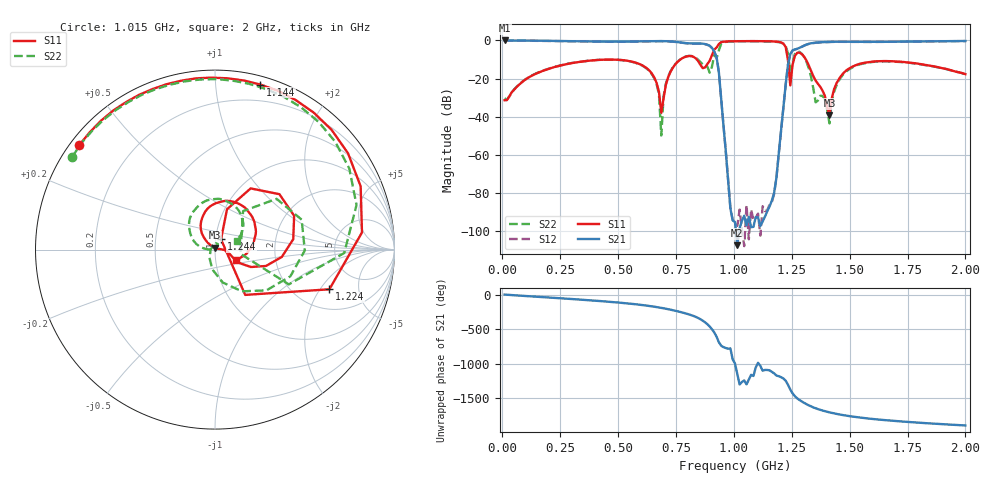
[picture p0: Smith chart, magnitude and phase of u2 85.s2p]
!Agilent Technologies,E8363B,SG43030131,A.07.50.48
!Agilent E8363B: A.07.50.48
!Date: Tuesday, December 02, 2025 02:39:29
!Correction: S11(Full 2 Port(1,2))
!S21(Full 2 Port(1,2))
!S12(Full 2 Port(1,2))
!S22(Full 2 Port(1,2))
!S2P File: Measurements: S11, S21, S12, S22:
# Hz S  dB  R 50
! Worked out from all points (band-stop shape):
!   201 points, 10 MHz to 2 GHz, reference 50 ohm
!   highest |S21| = -0.01 dB at 10 MHz (marker M1); lowest = -107.4 dB at 1.015 GHz (marker M2)
!   |S21| within 3 dB of the highest: start of sweep to 897.6 MHz; 1.298 GHz to end of sweep
!   lowest |S11| = -39.3 dB at 1.413 GHz (marker M3), VSWR 1.02, Z = 49.8 + j1.07 ohm
!   |S11| at or under -10 dB: start of sweep to 769.2 MHz; 839.9 MHz to 897.7 MHz (57.8 MHz wide, 6.65 % of centre); 1.311 GHz to end of sweep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
!   |S22| runs from -49.9 to -0.4 dB; largest |S21 - S12| = 0.028
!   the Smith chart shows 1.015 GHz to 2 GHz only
!   S11 on the Smith chart (normalised r, x): 1.015 GHz: 0.03, +0.34; 1.144 GHz: 0.06, +1.31; 1.224 GHz: 3.02, -2.45; 1.244 GHz: 1.06, +0.12; 2 GHz: 1.25, -0.15
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1e7  -31.35 -84.1  -0.01 -0.2  -0.08 -1.8  -30.31 -82.0
3.483e8  -11.00 -166.0  -0.48 -76.0  -0.56 -76.1  -10.98 -163.0
6.7665e8  -26.97 90.9  -0.33 173.4  -0.40 173.2  -28.39 86.0
6.866e8  -37.97 119.2  -0.34 167.5  -0.40 167.5  -49.85 63.0
6.9655e8  -30.37 -131.6  -0.36 161.5  -0.42 161.4  -29.29 -103.2
7.264e8  -16.44 -138.1  -0.51 141.4  -0.58 141.3  -16.21 -123.5
8.5575e8  -12.78 57.2  -1.60 3.4  -1.67 3.2  -11.41 141.5
8.856e8  -12.44 -74.1  -2.25 -68.4  -2.30 -68.6  -13.63 125.3
9.1545e8  -4.79 -116.6  -5.87 172.2  -5.93 172.0  -7.67 -104.3
9.7515e8  -0.49 169.0  -73.45 -62.2  -72.79 -47.4  -0.63 176.2
1.005e9  -0.42 148.3  -95.23 83.7  -94.76 66.1  -0.47 153.2
1.01495e9  -0.40 142.5  -107.36 -69.8  -97.25 142.5  -0.45 147.0
1.1443e9  -0.41 74.6  -89.59 -9.3  -89.12 -89.0  -0.51 78.5
1.17415e9  -0.53 54.3  -79.77 -59.0  -80.40 -41.9  -0.66 58.9
1.2239e9  -3.42 -19.1  -23.12 -164.7  -23.18 -164.9  -2.85 -1.5
1.2438e9  -23.57 59.6  -7.14 68.5  -7.19 68.4  -16.85 -9.4
1.29355e9  -7.13 7.6  -3.27 -104.8  -3.34 -104.9  -7.03 -19.6
1.3433e9  -18.78 -25.3  -1.30 170.6  -1.37 170.5  -25.20 -124.3
1.41295e9  -39.25 99.4  -0.76 99.0  -0.82 98.9  -43.50 145.3
1.47265e9  -17.22 125.0  -0.67 58.7  -0.73 58.6  -17.78 157.5
1.67165e9  -10.82 54.7  -0.69 -18.7  -0.75 -18.9  -11.00 82.1
2e9  -17.70 -26.9  -0.29 -90.2  -0.35 -90.4  -17.77 22.1
